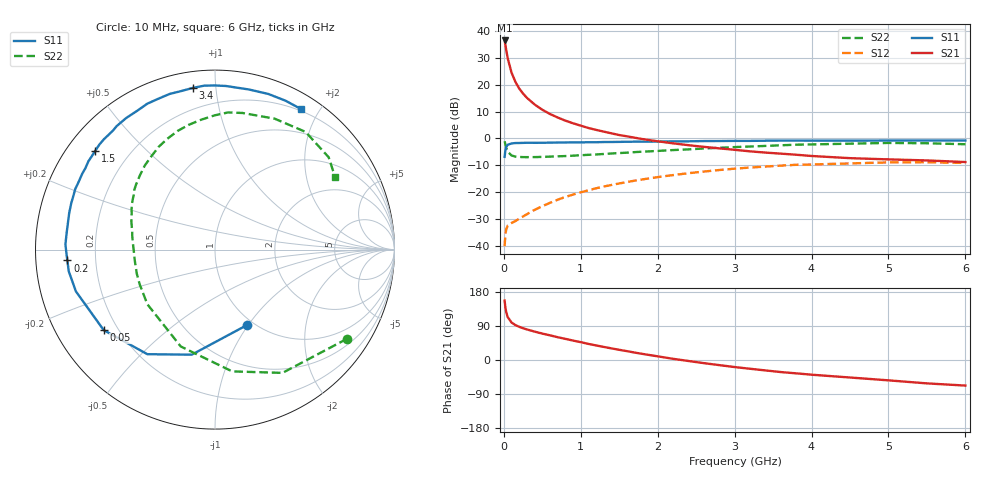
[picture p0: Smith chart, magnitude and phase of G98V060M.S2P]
! SIEMENS Small Signal Semiconductors
! BFG235
! Si NPN RF Bipolar Junction Transistor in SOT223
! VCE = 8 V  IC = 60 mA
! Common Emitter S-Parameters:  July  1994
# GHz  S  MA  R  50
!  f  S11  S21  S12  S22
! GHz  MAG  ANG  MAG  ANG  MAG  ANG  MAG  ANG
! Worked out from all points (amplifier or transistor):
!   40 points, 10 MHz to 6 GHz, reference 50 ohm
!   highest |S21| = 36.3 dB at 10 MHz (marker M1)
!   |S21| within 3 dB of that: start of sweep to 27.9 MHz
!   unconditionally stable (mu >= 1): 492.8 MHz to 1.288 GHz
!   at 200 MHz: K = 0.70, MSG = 24.1 dB, |S12| = -29.7 dB
!   at 1.5 GHz: K = 0.98, MSG = 9.0 dB, |S12| = -16.7 dB
!   at 6 GHz: K = 0.91, MSG = 0.2 dB, |S12| = -9.1 dB
!   S11 on the Smith chart (normalised r, x): 10 MHz: 0.93, -0.99; 50 MHz: 0.15, -0.32; 200 MHz: 0.10, -0.04; 1.5 GHz: 0.08, +0.36; 3.4 GHz: 0.08, +0.87; 6 GHz: 0.18, +1.76
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0.01  0.4565 -66.7  65.61 156.7  0.0101 68.9  0.8879 -34.0
0.02  0.5997 -102.5  54.29 139.2  0.0164 53.3  0.7831 -61.3
0.03  0.694 -122.9  44.57 127.1  0.0205 44.5  0.6852 -82.0
0.05  0.7654 -144.1  30.78 113.2  0.0243 34.6  0.5724 -109.5
0.1  0.8093 -163.3  16.64 99.0  0.0271 31.8  0.4845 -141.1
0.15  0.8235 -171.5  11.23 92.1  0.0295 35.4  0.4621 -155.2
0.2  0.825 -175.8  8.424 87.6  0.0327 39.2  0.4558 -163.1
0.25  0.8293 -179.4  6.79 83.8  0.0359 42.4  0.4516 -168.3
0.3  0.8339 177.9  5.67 80.7  0.0395 45.9  0.4511 -172.4
0.4  0.8317 173.1  4.268 74.9  0.0476 49.7  0.4518 -178.0
0.5  0.8332 169.2  3.407 69.7  0.0556 52.5  0.456 177.7
0.6  0.8375 165.9  2.842 65.1  0.0642 53.5  0.4614 173.9
0.7  0.8416 162.1  2.448 60.1  0.0734 54.3  0.4674 170.6
0.9  0.8486 156.6  1.913 51.3  0.0913 53.1  0.4803 164.8
1.1  0.8522 150.1  1.564 42.4  0.1099 51.0  0.4984 159.2
1.5  0.8651 140.4  1.159 26.9  0.1468 44.8  0.5373 148.5
2.2  0.8845 124.0  0.813 3.1  0.2099 30.6  0.6105 129.8
3.2  0.903 102.2  0.578 -23.1  0.2894 7.2  0.71 102.0
3.4  0.9095 97.7  0.548 -27.5  0.3018 2.2  0.7281 96.0
4.5  0.9119 78.0  0.432 -46.2  0.3452 -23.8  0.8016 65.5
5.5  0.9179 64.7  0.392 -61.7  0.3633 -46.2  0.816 39.1
6  0.918 58.7  0.366 -67.5  0.3523 -54.7  0.7823 31.3
